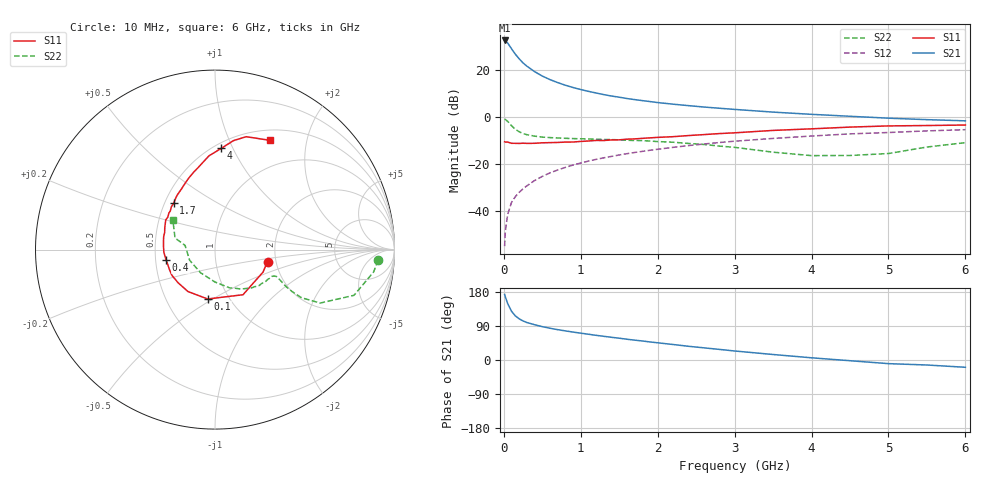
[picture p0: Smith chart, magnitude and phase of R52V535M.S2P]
! SIEMENS Small Signal Semiconductors
! BFR183
! Si NPN RF Bipolar Junction Transistor in SOT23
! VCE = 2.5 V  IC = 35 mA
! Common Emitter S-Parameters:  May  1996
# GHz  S  MA  R  50
!  f  S11  S21  S12  S22
! GHz  MAG  ANG  MAG  ANG  MAG  ANG  MAG  ANG
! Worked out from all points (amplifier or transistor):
!   36 points, 10 MHz to 6 GHz, reference 50 ohm
!   highest |S21| = 32.7 dB at 10 MHz (marker M1)
!   |S21| within 3 dB of that: start of sweep to 89.02 MHz
!   unconditionally stable (mu >= 1): start of sweep to 10.27 MHz; 322.6 MHz to 2.417 GHz
!   at 250 MHz: K = 0.95, MSG = 26.8 dB, |S12| = -30.5 dB
!   at 1.4 GHz: K = 1.06, MAG = 11.3 dB, |S12| = -16.7 dB
!   at 6 GHz: K = 0.92, MSG = 1.9 dB, |S12| = -5.3 dB
!   S11 on the Smith chart (normalised r, x): 10 MHz: 1.80, -0.27; 100 MHz: 0.80, -0.48; 400 MHz: 0.57, -0.07; 1.7 GHz: 0.56, +0.33; 4 GHz: 0.54, +0.90; 6 GHz: 0.63, +1.43
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0.01  0.3001 -12.9  42.97 173.1  0.0018 84.1  0.9109 -3.7
0.02  0.2955 -25.2  42.19 166.3  0.0038 82.7  0.8926 -8.0
0.05  0.2958 -58.2  37.87 148.9  0.0086 76.3  0.8155 -18.2
0.1  0.2782 -98.4  28.6 128.8  0.0154 71.5  0.6579 -26.9
0.15  0.2779 -122.7  21.86 116.2  0.0204 69.4  0.5522 -29.1
0.2  0.2765 -137.9  17.44 108.6  0.0252 71.1  0.4899 -28.6
0.25  0.2795 -148.9  14.29 103.0  0.03 72.1  0.4495 -27.6
0.3  0.2772 -155.9  12.16 98.9  0.0347 73.8  0.424 -26.4
0.4  0.2783 -168.0  9.331 93.1  0.0449 74.1  0.3953 -24.8
0.5  0.2853 -176.9  7.507 88.0  0.055 75.0  0.3774 -23.8
0.6  0.2875 176.5  6.308 83.8  0.0653 74.4  0.368 -23.7
0.7  0.2902 171.5  5.453 80.1  0.0753 74.2  0.3614 -24.1
0.9  0.2963 161.2  4.283 73.7  0.096 72.8  0.3506 -25.2
1.1  0.3115 153.0  3.546 68.0  0.1164 71.1  0.3435 -27.9
1.4  0.3279 141.5  2.819 59.9  0.1465 68.1  0.3339 -32.0
1.7  0.3455 131.7  2.368 52.4  0.1774 64.9  0.3197 -36.9
2.2  0.3851 119.2  1.893 40.9  0.2283 58.9  0.2934 -47.1
3.5  0.5233 93.7  1.283 14.5  0.3533 41.4  0.1801 -90.4
4  0.5656 86.4  1.151 5.8  0.3975 35.1  0.1521 -122.0
4.5  0.6157 80.4  1.046 -1.9  0.4415 28.1  0.1532 -157.3
5.5  0.6649 68.4  0.887 -13.2  0.5113 15.9  0.2318 163.9
6  0.6814 63.3  0.837 -19.2  0.5426 8.2  0.2874 144.8
